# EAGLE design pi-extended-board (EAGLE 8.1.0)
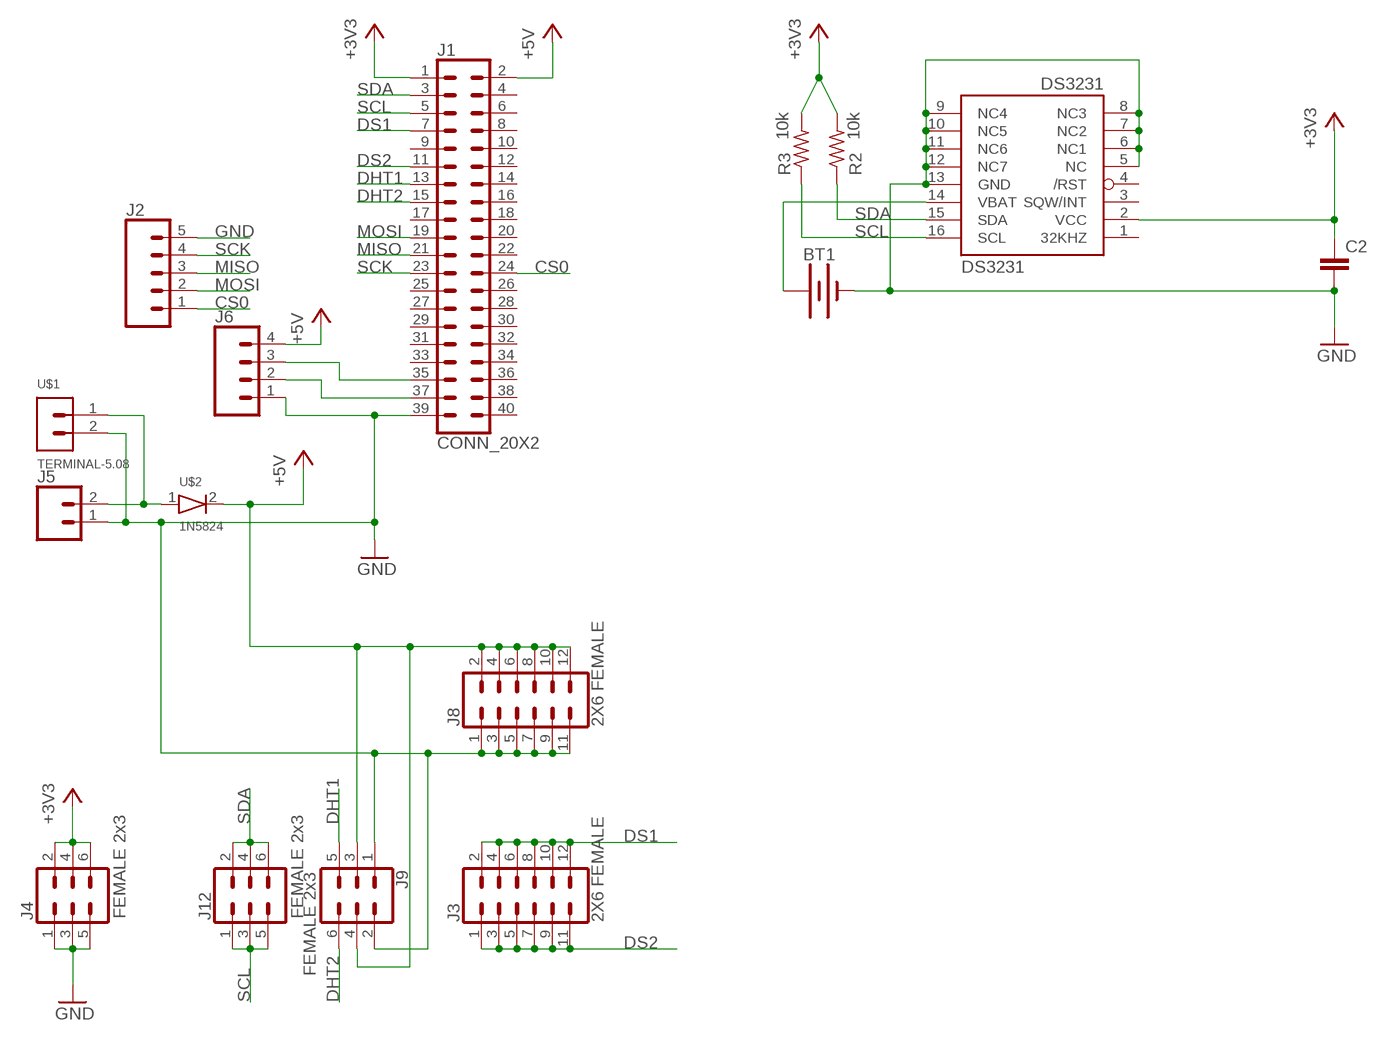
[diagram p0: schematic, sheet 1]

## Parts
BT1  BATTERY-20MM_PTH  [BATTCOM_20MM_PTH]
C2  C-EUC0805  [C0805]
DS3231  DS3231/SO  [SO16W]
J1  CONN_20X2  [2X20]
J2  CONN_05KH2510  [1X05KF2510]
J3  2X6 FEMALE  CONN_06X2PTH_FEMALE  [2X6]
J4  FEMALE 2x3  CONN_03X2FEMALE  [2X3]
J5  CONN_02POLAR  [MOLEX-1X2]
J6  CONN_04POLAR  [MOLEX-1X4]
J8  2X6 FEMALE  CONN_06X2PTH_FEMALE  [2X6]
J9  FEMALE 2x3  CONN_03X2FEMALE  [2X3]
J12  FEMALE 2x3  CONN_03X2FEMALE  [2X3]
R2  10k  R-US_R0805  [R0805]
R3  10k  R-US_R0805  [R0805]
U$1  TERMINAL-5.08  [TERMINAL-5.08]
U$2  1N5824  [DIODE-1N5824,SMD]

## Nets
+3V3: C2.1 DS3231.2(VCC) J1.1 J4.2 J4.4 J4.6 R2.2 R3.2
+5V: J1.2 J6.4 J8.2 J8.4 J8.6 J8.8 J8.10 J8.12 J9.3 J9.4 U$2.2
CS0: J1.24 J2.1
DHT1: J1.13 J9.5
DHT2: J1.15 J9.6
DS1: J1.7 J3.2 J3.4 J3.6 J3.8 J3.10 J3.12
DS2: J1.11 J3.1 J3.3 J3.5 J3.7 J3.9 J3.11
GND: BT1.2(-) C2.2 DS3231.5(NC) DS3231.6(NC1) DS3231.7(NC2) DS3231.8(NC3) DS3231.9(NC4) DS3231.10(NC5) DS3231.11(NC6) DS3231.12(NC7) DS3231.13(GND) J1.39 J2.5 J4.1 J4.3 J4.5 J5.1 J6.1 J8.1 J8.3 J8.5 J8.7 J8.9 J8.11 J9.1 J9.2 U$1.2
MISO: J1.21 J2.3
MOSI: J1.19 J2.2
N$1: J5.2 U$1.1 U$2.1
N$2: BT1.1(+) DS3231.14(VBAT)
N$3: J1.37 J6.2
N$4: J1.35 J6.3
SCK: J1.23 J2.4
SCL: DS3231.16(SCL) J1.5 J12.1 J12.3 J12.5 R3.1
SDA: DS3231.15(SDA) J1.3 J12.2 J12.4 J12.6 R2.1
Unconnected: DS3231.1(32KHZ) DS3231.3(SQW/INT) DS3231.4(/RST) J1.4 J1.6 J1.8 J1.9 J1.10 J1.12 J1.14 J1.16 J1.17 J1.18 J1.20 J1.22 J1.25 J1.26 J1.27 J1.28 J1.29 J1.30 J1.31 J1.32 J1.33 J1.34 J1.36 J1.38 J1.40

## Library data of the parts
BT1 = SparkFun-Batteries:BATTERY: Battery - Single Cell; PROD_ID: BATT-09031; SF_SKU: PRT-00783
C2 = resistor:C-EU: CAPACITOR, European symbol
DS3231 = adafruit:DS3231
J1 = SparkFun-Connectors:CONN_20X2: Multi connection point. Often used as Generic Header-pin footprint for 0.1 inch spaced/style header connections On any of the 0.1 inch spaced packages, you can populate with these: Break Away Headers - Straight (PRT-00116) Break Away Male Headers - Right Angle (PRT-00553) Female Headers (PRT-00115)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
J2 = bon-connecters:CONN_05: Multi connection point. Often used as Generic Header-pin footprint for 0.1 inch spaced/style header connections On any of the 0.1 inch spaced packages, you can populate with these: Break Away Headers - Straight (PRT-00116) Break Away Male Headers - Right Angle (PRT-00553) Female Headers (PRT-00115)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
J3 J8 = SparkFun-Connectors:CONN_06X2: Multi connection point. Often used as Generic Header-pin footprint for 0.1 inch spaced/style header connections On any of the 0.1 inch spaced packages, you can populate with these: Break Away Headers - Straight (PRT-00116) Break Away Male Headers - Right Angle (PRT-00553) Female Headers (PRT-00115)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; PROD_ID: CONN-12423
J4 J9 J12 = SparkFun-Connectors:CONN_03X2: Multi connection point. Often used as Generic Header-pin footprint for 0.1 inch spaced/style header connections You can populate with any combo of single row headers, but if you'd like an exact match, check these: Header - 2x3 (Male, 0.1") (PRT-12807) Header - 2x3 (Female, 0.1") (PRT-13010) 2x3 Pin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; PROD_ID: CONN-11566
J5 = SparkFun-Connectors:CONN_02: Multi connection point. Often used as Generic Header-pin footprint for 0.1 inch spaced/style header connections; SF_ID: PRT-09918
J6 = SparkFun-Connectors:CONN_04: Multi connection point. Often used as Generic Header-pin footprint for 0.1 inch spaced/style header connections On any of the 0.1 inch spaced packages, you can populate with these: Break Away Headers - Straight (PRT-00116) Break Away Male Headers - Right Angle (PRT-00553) Female Headers (PRT-00115)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; PROD_ID: CONN-08186; SF_ID: PRT-08231
R2 R3 = adafruit:R-US_: RESISTOR, American symbol
U$1 = huike:TERMINAL-5.08
U$2 = huike:1N5824

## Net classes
0 +5V: width 0.61 mm, drill 0.61 mm, clearance 0.61 mm

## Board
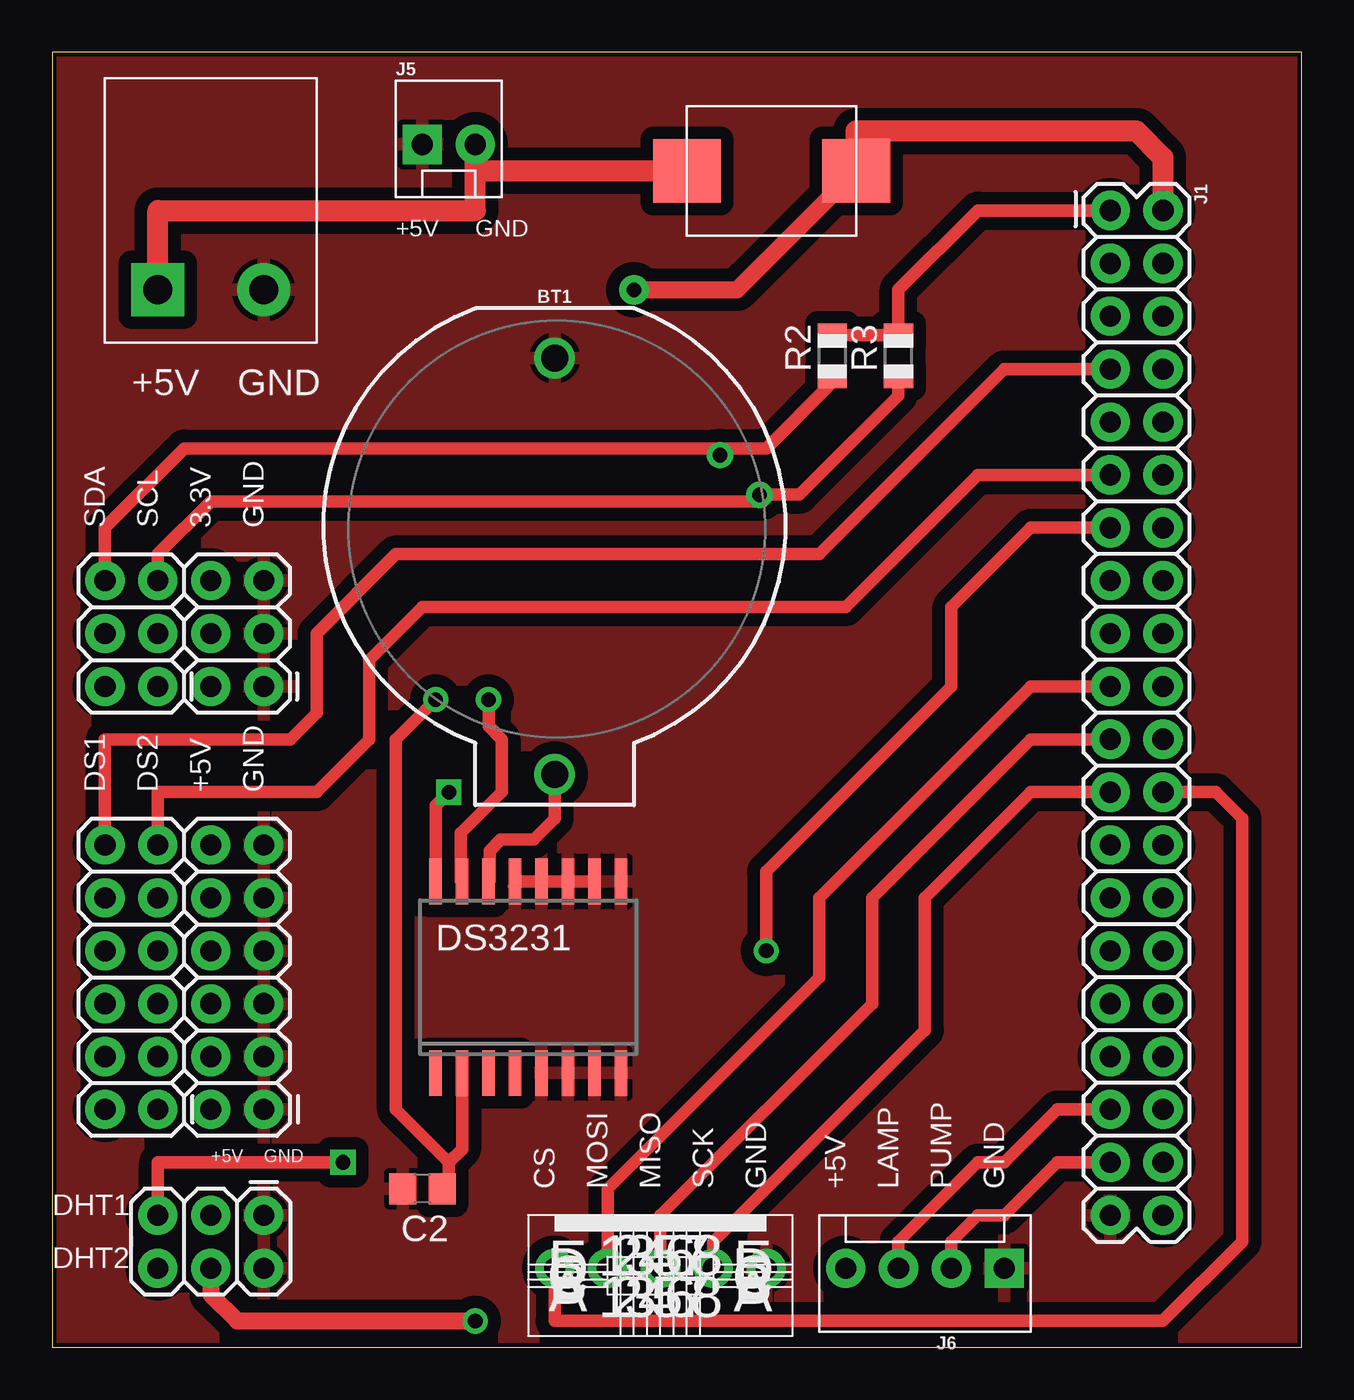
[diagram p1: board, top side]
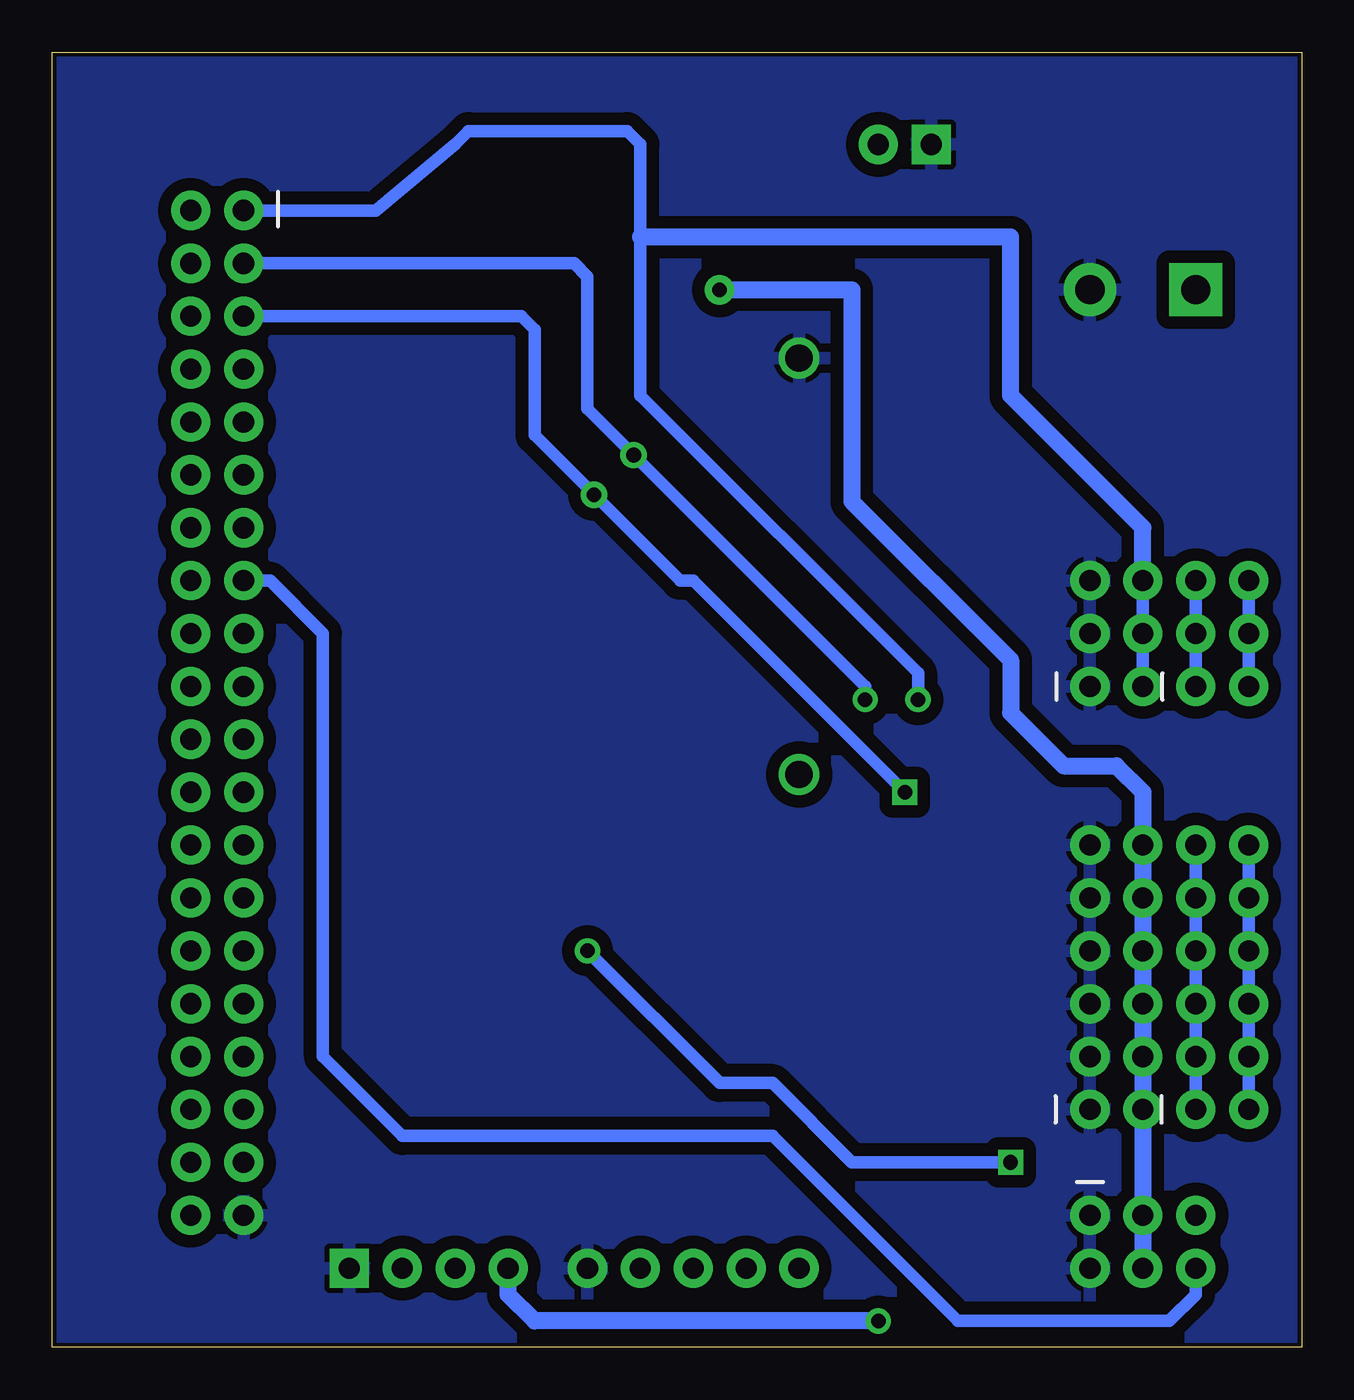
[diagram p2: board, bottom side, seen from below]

Size 59.99 x 62.22 mm. Coordinates in mm from the lower left corner, seen from the top.
Outline: 0,0 59.99,0 59.99,62.22 0,62.22 0,0
Copper layers (1*16): Top 0.035mm / dielectric 1.5mm / Bottom 0.035mm
Design rules "SparkFun": minimum track width 8mil, minimum drill 20mil, track to track 8mil, track to pad 8mil, pad to pad 8mil, via to via 8mil, smd to smd 8mil, copper to edge 8mil, drill to drill 8mil, minimum pad ring 12mil, minimum via ring 10mil, stop-mask expansion 4mil, vias tented up to drill 20mil, thermal gap 10mil

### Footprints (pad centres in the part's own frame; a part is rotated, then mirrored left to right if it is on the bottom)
BATTCOM_20MM_PTH = drill 1.3: 1 11.85,0; 2 -8.15,0
C0805 = smd 1.3 x 1.5: 1 -0.95,0; 2 0.95,0
SO16W = smd 0.6 x 2.2: 1 -4.445,-4.6; 2 -3.175,-4.6; 3 -1.905,-4.6; 4 -0.635,-4.6; 5 0.635,-4.6; 6 1.905,-4.6; 7 3.175,-4.6; 8 4.445,-4.6; 9 4.445,4.6; 10 3.175,4.6; 11 1.905,4.6; 12 0.635,4.6; 13 -0.635,4.6; 14 -1.905,4.6; 15 -3.175,4.6; 16 -4.445,4.6
2X20 = drill 1.016 pad 1.88: 1 0,0; 2 0,2.54; 3 2.54,0; 4 2.54,2.54; 5 5.08,0; 6 5.08,2.54; 7 7.62,0; 8 7.62,2.54; 9 10.16,0; 10 10.16,2.54; 11 12.7,0; 12 12.7,2.54; 13 15.24,0; 14 15.24,2.54; 15 17.78,0; 16 17.78,2.54; 17 20.32,0; 18 20.32,2.54; 19 22.86,0; 20 22.86,2.54; 21 25.4,0; 22 25.4,2.54; 23 27.94,0; 24 27.94,2.54; 25 30.48,0; 26 30.48,2.54; 27 33.02,0; 28 33.02,2.54; 29 35.56,0; 30 35.56,2.54; 31 38.1,0; 32 38.1,2.54; 33 40.64,0; 34 40.64,2.54; 35 43.18,0; 36 43.18,2.54; 37 45.72,0; 38 45.72,2.54; 39 48.26,0; 40 48.26,2.54
1X05KF2510 = drill 1.016 pad 1.88: 1 0,0; 2 2.54,0; 3 5.08,0; 4 7.62,0; 5 10.16,0
2X6 = drill 1.016 pad 1.88: 1 0,0; 2 0,2.54; 3 2.54,0; 4 2.54,2.54; 5 5.08,0; 6 5.08,2.54; 7 7.62,0; 8 7.62,2.54; 9 10.16,0; 10 10.16,2.54; 11 12.7,0; 12 12.7,2.54
2X3 = drill 1.016 pad 1.88: 1 0,0; 2 0,2.54; 3 2.54,0; 4 2.54,2.54; 5 5.08,0; 6 5.08,2.54
MOLEX-1X2 = drill 1.016 pad 1.88 square: 1 0,0 | drill 1.016 pad 1.88: 2 2.54,0
MOLEX-1X4 = drill 1.016 pad 1.88 square: 1 0,0 | drill 1.016 pad 1.88: 2 2.54,0; 3 5.08,0; 4 7.62,0
R0805 = smd 1.1 x 1.4: 1 -1,0; 2 1,0
TERMINAL-5.08 = drill 1.4 pad 2.54 square: 1 0,0 | drill 1.4 pad 2.54: 2 5.08,0
DIODE-1N5824,SMD = smd 3.251 x 3.048: 1 0,0; 2 8.128,0

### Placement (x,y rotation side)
BT1  24.13,39.37 270 top
C2  17.78,7.62 180 top
DS3231  22.86,17.78 0 top
J1  50.8,54.61 270 top
J2  24.13,3.81 0 top
J3  5.08,11.43 90 top
J4  10.16,31.75 90 top
J5  17.78,57.78 0 top
J6  45.72,3.81 180 top
J8  10.16,11.43 90 top
J9  10.16,6.35 180 top
J12  5.08,31.75 90 top
R2  37.47,47.62 90 top
R3  40.64,47.62 90 top
U$1  5.08,50.8 0 top
U$2  30.48,56.52 0 top

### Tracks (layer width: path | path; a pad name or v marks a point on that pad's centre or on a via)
+3V3  (via drill 0.7)
  Top 0.61: 19.05,8.89 16.51,11.43 16.51,29.21 v18.41,31.11 | 19.05,8.89 19.05,7.94 C2.1 19.05,7.3 | R2.2 R3.2 40.64,50.8 44.45,54.61 J1.1 | DS3231.2 19.68,9.53 19.05,8.89
  Bottom 0.61: v18.41,31.11 18.41,32.38 31.75,45.72 31.75,53.34 31.75,57.78 32.38,58.42 40.01,58.42 40.64,57.78 44.45,54.61 J1.1 | J4.6 J4.4 J4.2
  Bottom 0.813: J4.6 7.62,39.37 13.97,45.72 13.97,53.34 31.75,53.34
+5V  (via drill 0.7, 0.7 pad 1.42)
  Top 0.813: v27.94,50.8 32.89,50.8 U$2.2 | J9.4 7.62,2.54 8.89,1.27 v20.32,1.27
  Top 1.016: J1.2 53.34,57.15 52.07,58.42 38.61,58.42 U$2.2
  Bottom 0.813: v27.94,50.8 21.59,50.8 21.59,40.64 13.97,33.02 13.97,30.48 11.43,27.94 8.89,27.94 7.62,26.67 J8.12 J8.10 J8.8 J8.6 J8.4 J8.2 J9.3 J9.4 | v20.32,1.27 36.83,1.27 38.1,2.54 J6.4
CS0
  Top 0.61: J1.24 55.88,26.67 57.15,25.4 57.15,5.08 53.34,1.27 24.13,1.27 J2.1
DHT1  (via drill 0.7)
  Top 0.61: J1.13 46.99,39.37 43.18,35.56 43.18,31.75 34.29,22.86 v34.29,19.05 | J9.5 5.08,8.89 v13.97,8.89
  Bottom 0.61: v34.29,19.05 27.94,12.7 25.4,12.7 21.59,8.89 v13.97,8.89
DHT2
  Bottom 0.61: J9.6 5.08,2.54 6.35,1.27 16.51,1.27 25.4,10.16 43.18,10.16 46.99,13.97 46.99,34.29 49.53,36.83 J1.15
DS1
  Top 0.61: J1.7 45.72,46.99 36.83,38.1 16.51,38.1 12.7,34.29 12.7,30.48 11.43,29.21 2.54,29.21 J3.12
  Bottom 0.61: J3.12 J3.10 J3.8 J3.6 J3.4 J3.2
DS2
  Top 0.61: J1.11 44.45,41.91 38.1,35.56 17.78,35.56 15.24,33.02 15.24,29.21 12.7,26.67 5.08,26.67 J3.11
  Bottom 0.61: J3.1 J3.3 J3.5 J3.7 J3.9 J3.11
GND
  Top 0.61: DS3231.13 DS3231.12 DS3231.11 DS3231.10
  pour Top: 0,0 0,62.23 59.69,62.23 59.69,0
  pour Bottom: 0,0 0,62.23 59.69,62.23 59.69,0
MISO
  Top 0.61: J1.21 46.99,29.21 39.37,21.59 39.37,16.51 29.21,6.35 J2.3
MOSI
  Top 0.61: J1.19 46.99,31.75 36.83,21.59 36.83,17.78 26.67,7.62 J2.2
N$1
  Top 1.016: 20.32,56.52 U$2.1 | 20.32,56.52 J5.2 | U$1.1 5.08,54.61 20.32,54.61 20.32,56.52
N$2
  Top 0.61: DS3231.14 21.01,22.43 21.01,23.85 21.55,24.39 23.12,24.39 24.13,25.4 BT1.1
N$3
  Top 0.61: J6.2 43.18,5.08 44.45,6.35 45.72,6.35 48.26,8.89 J1.37
N$4
  Top 0.61: J6.3 40.64,5.08 44.45,8.89 45.72,8.89 48.26,11.43 J1.35
SCK
  Top 0.61: J1.23 46.99,26.67 41.91,21.59 41.91,15.24 31.75,5.08 J2.4
SCL  (via drill 0.7, 0.7 pad 1.27)
  Top 0.61: J12.5 5.08,38.1 7.62,40.64 33.66,40.64 v33.97,40.96 35.88,40.96 40.64,45.72 R3.1 | DS3231.16 18.41,26.04 v19.05,26.67
  Bottom 0.61: J1.5 37.47,49.53 36.83,48.9 36.83,43.81 v33.97,40.96 29.84,36.83 29.21,36.83 v19.05,26.67 | J12.1 J12.3 J12.5
SDA  (via drill 0.7, 0.7 pad 1.27)
  Top 0.61: J12.6 2.54,39.37 6.35,43.18 31.75,43.18 v32.07,42.86 32.38,43.18 34.29,43.18 37.47,46.35 R2.1 | v20.95,31.11 20.95,29.84 21.59,29.21 21.59,26.67 19.63,24.71 19.63,22.43 DS3231.15
  Bottom 0.61: J1.3 34.92,52.07 34.29,51.44 34.29,45.09 v32.07,42.86 20.95,31.75 v20.95,31.11 | J12.6 J12.4 J12.2

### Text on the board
tNames: +5V | GND | +5V | GND | SDA | SCL | 3.3V | GND | DS1 | DS2 | +5V | GND | +5V | GND | CS | MOSI | MISO | SCK | GND | +5V | LAMP | PUMP | GND | DHT1 | DHT2
Document: DS1 | DS2 | +5V | GND | SDA | SCL | DHT1 | DHT2

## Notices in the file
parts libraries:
SparkFun-Batteries: Licensing: Creative Commons ShareAlike 4.0 International - https://creativecommons.org/licenses/by-sa/4.0
